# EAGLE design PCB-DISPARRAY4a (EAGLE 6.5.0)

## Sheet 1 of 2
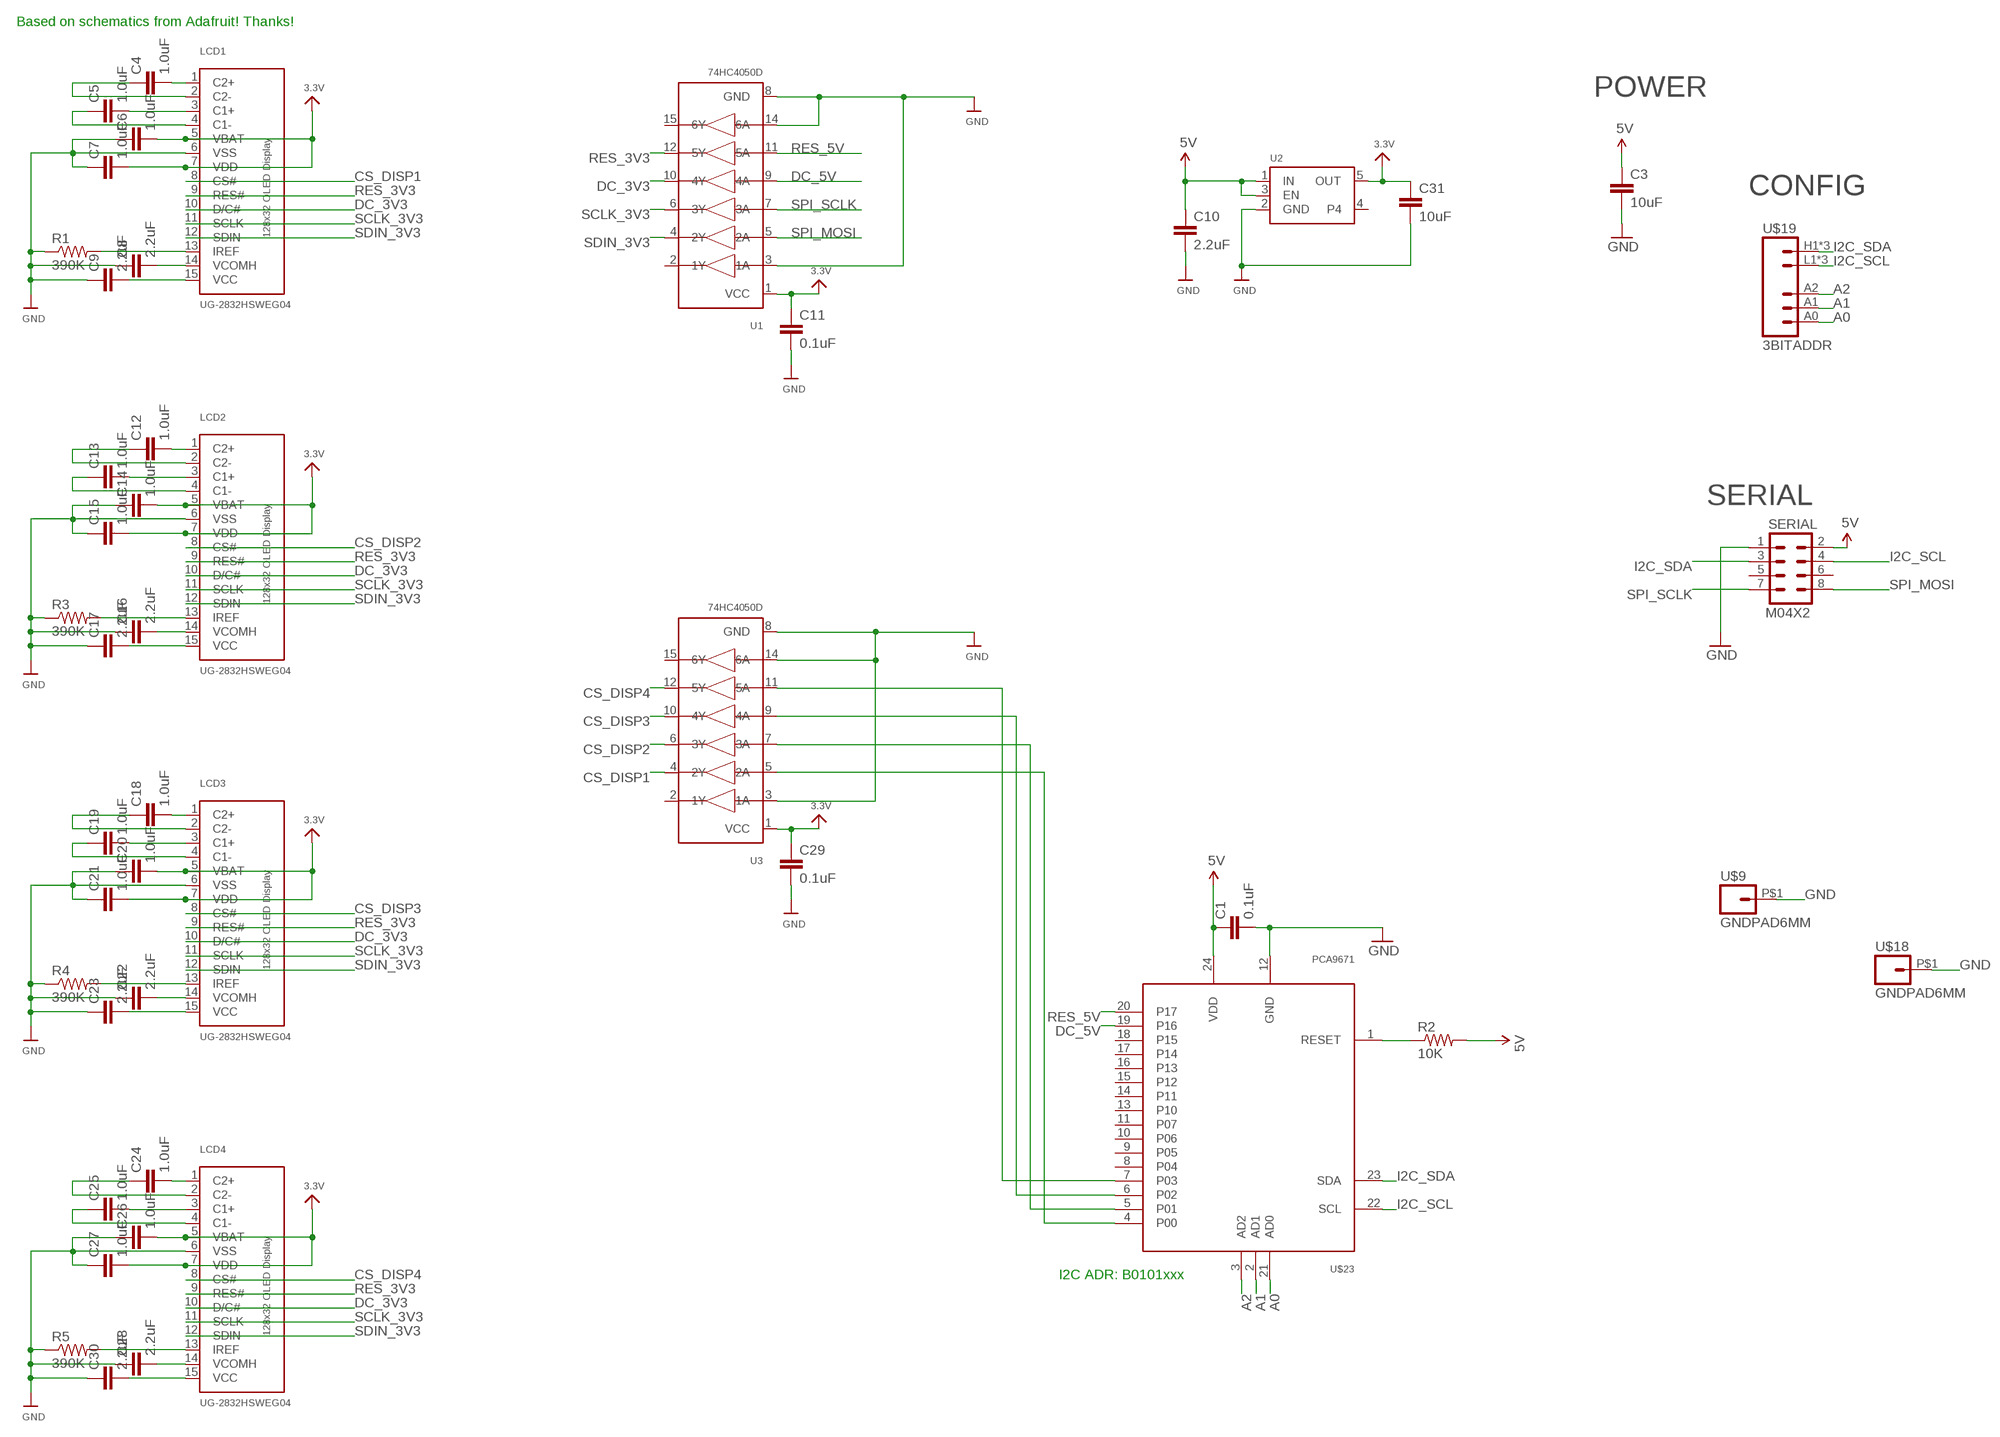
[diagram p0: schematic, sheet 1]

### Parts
C1  0.1uF  CAP0603-CAP  [0603-CAP]
C3  10uF  CAP0805  [0805]
C4  1.0uF  CAP0603-CAP  [0603-CAP]
C5  1.0uF  CAP0603-CAP  [0603-CAP]
C6  1.0uF  CAP0603-CAP  [0603-CAP]
C7  1.0uF  CAP0603-CAP  [0603-CAP]
C8  2.2uF  CAP0603-CAP  [0603-CAP]
C9  2.2uF  CAP0603-CAP  [0603-CAP]
C10  2.2uF  CAP0805  [0805]
C11  0.1uF  CAP0603-CAP  [0603-CAP]
C12  1.0uF  CAP0603-CAP  [0603-CAP]
C13  1.0uF  CAP0603-CAP  [0603-CAP]
C14  1.0uF  CAP0603-CAP  [0603-CAP]
C15  1.0uF  CAP0603-CAP  [0603-CAP]
C16  2.2uF  CAP0603-CAP  [0603-CAP]
C17  2.2uF  CAP0603-CAP  [0603-CAP]
C18  1.0uF  CAP0603-CAP  [0603-CAP]
C19  1.0uF  CAP0603-CAP  [0603-CAP]
C20  1.0uF  CAP0603-CAP  [0603-CAP]
C21  1.0uF  CAP0603-CAP  [0603-CAP]
C22  2.2uF  CAP0603-CAP  [0603-CAP]
C23  2.2uF  CAP0603-CAP  [0603-CAP]
C24  1.0uF  CAP0603-CAP  [0603-CAP]
C25  1.0uF  CAP0603-CAP  [0603-CAP]
C26  1.0uF  CAP0603-CAP  [0603-CAP]
C27  1.0uF  CAP0603-CAP  [0603-CAP]
C28  2.2uF  CAP0603-CAP  [0603-CAP]
C29  0.1uF  CAP0603-CAP  [0603-CAP]
C30  2.2uF  CAP0603-CAP  [0603-CAP]
C31  10uF  CAP0805  [0805]
LCD1  UG-2832HSWEG04  OLED_UG-2832HSWEG04WRAPAROUND  [UG-2832HSWEG04_WRAPAROUND]
LCD2  UG-2832HSWEG04  OLED_UG-2832HSWEG04WRAPAROUND  [UG-2832HSWEG04_WRAPAROUND]
LCD3  UG-2832HSWEG04  OLED_UG-2832HSWEG04WRAPAROUND  [UG-2832HSWEG04_WRAPAROUND]
LCD4  UG-2832HSWEG04  OLED_UG-2832HSWEG04WRAPAROUND  [UG-2832HSWEG04_WRAPAROUND]
R1  390K  RESISTOR0603-RES  [0603-RES]
R2  10K  RESISTOR0603-RES  [0603-RES]
R3  390K  RESISTOR0603-RES  [0603-RES]
R4  390K  RESISTOR0603-RES  [0603-RES]
R5  390K  RESISTOR0603-RES  [0603-RES]
SERIAL  M04X2  [2X4]
U1  74HC4050D  74HC4050DTSSOP16  [TSSOP16]
U2  VREG_SOT23-5  [SOT23-5]
U3  74HC4050D  74HC4050DTSSOP16  [TSSOP16]
U$9  GNDPAD6MM  [3.2MMPAD6MM]
U$18  GNDPAD6MM  [3.2MMPAD6MM]
U$19  3BITADDR  [3BITADDR]
U$23  PCA9671  [TSSOP24]

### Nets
3.3V [Power]: C6.2 C7.2 C11.1 C14.2 C15.2 C20.2 C21.2 C26.2 C27.2 C29.1 C31.1 LCD1.5(VBAT) LCD1.7(VDD) LCD2.5(VBAT) LCD2.7(VDD) LCD3.5(VBAT) LCD3.7(VDD) LCD4.5(VBAT) LCD4.7(VDD) U1.1(VCC) U2.5(OUT) U3.1(VCC)
5V [Power]: C1.1 C3.1 C10.1 R2.2 SERIAL.2 U2.1(IN) U2.3(EN) U$23.24(VDD)
A0: U$19.A0 U$23.21(AD0)
A1: U$19.A1 U$23.2(AD1)
A2: U$19.A2 U$23.3(AD2)
CS_DISP1: LCD1.8(CS#) U3.4(2Y)
CS_DISP2: LCD2.8(CS#) U3.6(3Y)
CS_DISP3: LCD3.8(CS#) U3.10(4Y)
CS_DISP4: LCD4.8(CS#) U3.12(5Y)
DC_3V3: LCD1.10(D/C#) LCD2.10(D/C#) LCD3.10(D/C#) LCD4.10(D/C#) U1.10(4Y)
DC_5V: U1.9(4A) U$23.19(P16)
GND [Power]: C1.2 C3.2 C6.1 C7.1 C8.1 C9.1 C10.2 C11.2 C14.1 C15.1 C16.1 C17.1 C20.1 C21.1 C22.1 C23.1 C26.1 C27.1 C28.1 C29.2 C30.1 C31.2 LCD1.6(VSS) LCD2.6(VSS) LCD3.6(VSS) LCD4.6(VSS) R1.1 R3.1 R4.1 R5.1 SERIAL.1 U1.3(1A) U1.8(GND) U1.14(6A) U2.2(GND) U3.3(1A) U3.8(GND) U3.14(6A) U$9.P$1 U$18.P$1 U$23.12(GND)
I2C_SCL: SERIAL.4 U$19.L1(GND) U$19.L2(GND) U$19.L3(GND) U$23.22(SCL)
I2C_SDA: SERIAL.3 U$19.H1(VCC) U$19.H2(VCC) U$19.H3(VCC) U$23.23(SDA)
N$1: R2.1 U$23.1(RESET)
N$2: C4.1 LCD1.2(C2-)
N$3: C4.2 LCD1.1(C2+)
N$4: C5.1 LCD1.4(C1-)
N$5: C12.1 LCD2.2(C2-)
N$6: C12.2 LCD2.1(C2+)
N$7: C5.2 LCD1.3(C1+)
N$8: LCD1.13(IREF) R1.2
N$9: C8.2 LCD1.14(VCOMH)
N$10: C13.1 LCD2.4(C1-)
N$11: C13.2 LCD2.3(C1+)
N$12: LCD2.13(IREF) R3.2
N$13: C16.2 LCD2.14(VCOMH)
N$14: C17.2 LCD2.15(VCC)
N$15: C18.1 LCD3.2(C2-)
N$16: C18.2 LCD3.1(C2+)
N$17: C19.1 LCD3.4(C1-)
N$18: C19.2 LCD3.3(C1+)
N$19: LCD3.13(IREF) R4.2
N$20: C22.2 LCD3.14(VCOMH)
N$21: C23.2 LCD3.15(VCC)
N$22: C24.1 LCD4.2(C2-)
N$23: C24.2 LCD4.1(C2+)
N$24: C25.1 LCD4.4(C1-)
N$25: C25.2 LCD4.3(C1+)
N$26: LCD4.13(IREF) R5.2
N$27: C28.2 LCD4.14(VCOMH)
N$28: C9.2 LCD1.15(VCC)
N$29: U3.5(2A) U$23.4(P00)
N$30: U3.7(3A) U$23.5(P01)
N$31: U3.9(4A) U$23.6(P02)
N$32: U3.11(5A) U$23.7(P03)
N$33: C30.2 LCD4.15(VCC)
RES_3V3: LCD1.9(RES#) LCD2.9(RES#) LCD3.9(RES#) LCD4.9(RES#) U1.12(5Y)
RES_5V: U1.11(5A) U$23.20(P17)
SCLK_3V3: LCD1.11(SCLK) LCD2.11(SCLK) LCD3.11(SCLK) LCD4.11(SCLK) U1.6(3Y)
SDIN_3V3: LCD1.12(SDIN) LCD2.12(SDIN) LCD3.12(SDIN) LCD4.12(SDIN) U1.4(2Y)
SPI_MOSI: SERIAL.8 U1.5(2A)
SPI_SCLK: SERIAL.7 U1.7(3A)
Unconnected: SERIAL.5 SERIAL.6 U1.2(1Y) U1.15(6Y) U2.4 U3.2(1Y) U3.15(6Y) U$23.8(P04) U$23.9(P05) U$23.10(P06) U$23.11(P07) U$23.13(P10) U$23.14(P11) U$23.15(P12) U$23.16(P13) U$23.17(P14) U$23.18(P15)

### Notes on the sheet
- Based on schematics from Adafruit! Thanks!
- POWER
- CONFIG
- SERIAL
- I2C ADR: B0101xxx

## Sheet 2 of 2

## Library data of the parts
C1 C3-C31 = SparkFun:CAP: Capacitor
LCD1-LCD4 = microbuilder:OLED_UG-2832HSWEG04: 128x32 SPI 0.91" Monochrome OLED Display
R1-R5 = SparkFun:RESISTOR: Resistor
SERIAL = SparkFun:M04X2
U1 U3 = SKAARHOJ:74HC4050D: 6-channel level shifter 74HC4050D - 2V-6V Supply Digikey: 74HC4050D,653-ND Mouser: 771-74HC4050D-T
U2 = microbuilder:VREG_SOT23-5: SOT23-5 Fixed Voltage Regulators To better organise some of the SOT23-5 fixed voltage regulators in this library, this new part was created. Part Current Out V Out V In V Dropout Digikey Part No. ADP121 150mA 3.3V 3.4-5.5V 0.09V @ 150mA ADP121-AUJZ33R7CT-ND ADP121 150mA 3.0V 3.1-5.5V 0.09V @ 150mA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
U$9 U$18 = SKAARHOJ:GNDPAD
U$19 = SKAARHOJ:3BITADDR
U$23 = SKAARHOJ:PCA9671

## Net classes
0 default: width 0.203 mm, drill 0.406 mm, clearance 0.152 mm
1 Power: width 0.406 mm, drill 0.61 mm, clearance 0.203 mm

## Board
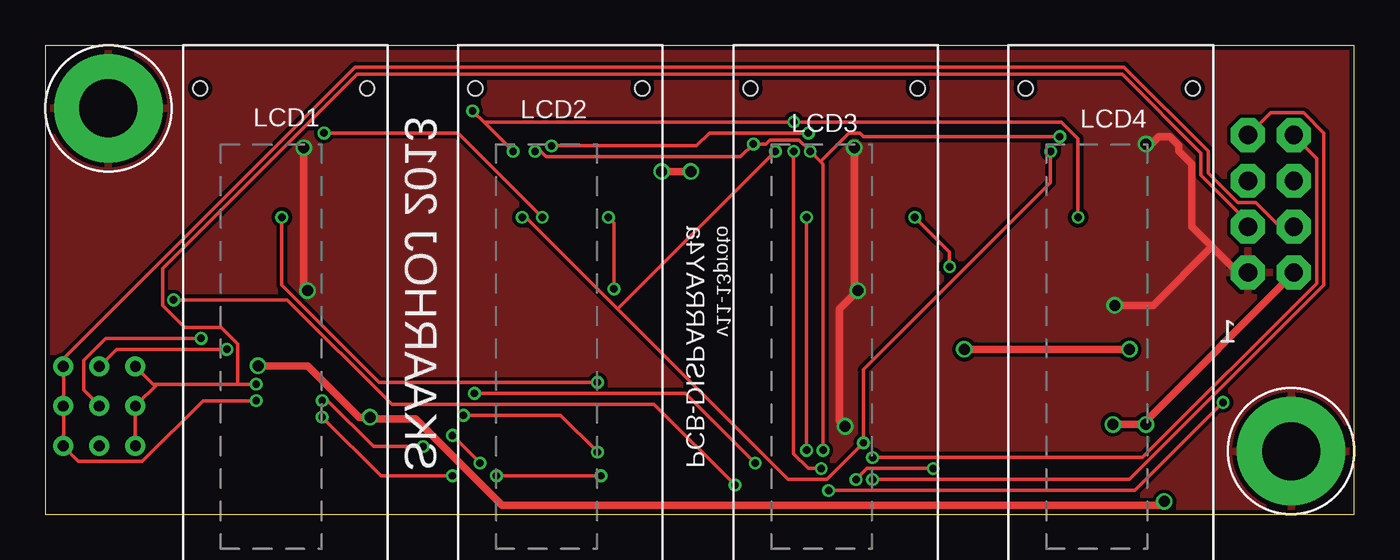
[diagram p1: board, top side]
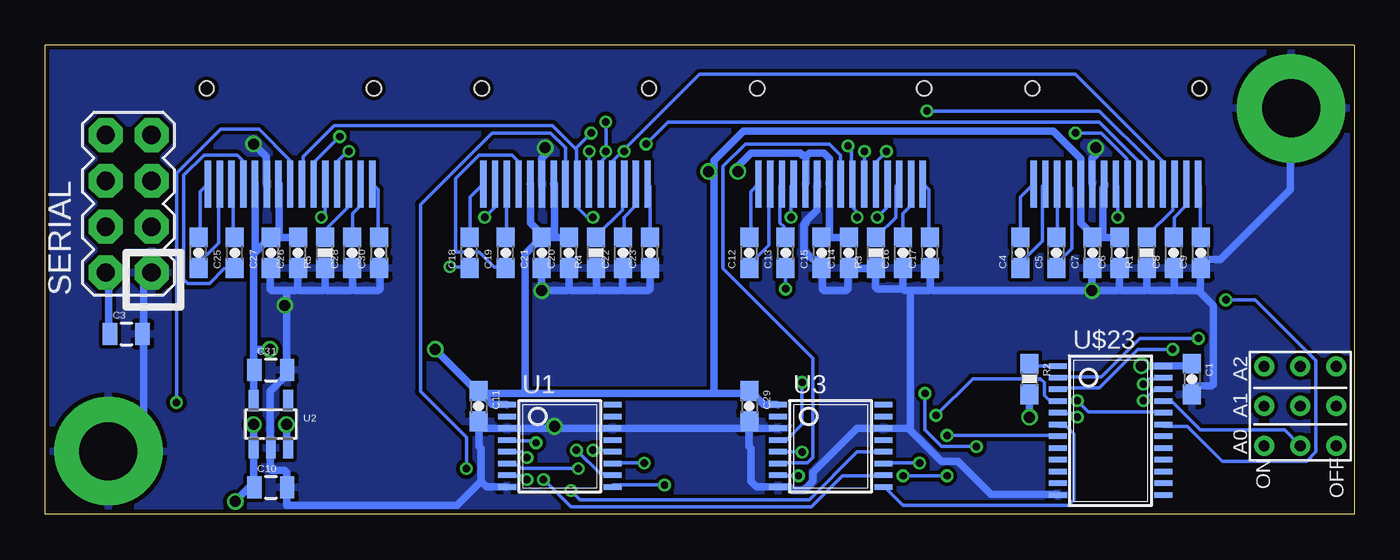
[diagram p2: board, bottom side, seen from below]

Size 72.5 x 26 mm. Coordinates in mm from the lower left corner, seen from the top.
Outline: 72.5,0 72.5,26 0,26 0,0 72.5,0
Copper layers (1*16): Top 0.035mm / dielectric 1.5mm / Bottom 0.035mm
Design rules "Fusion_eagle_rule_v1.1": minimum track width 6mil, minimum drill 12mil, track to track 6mil, track to pad 6mil, pad to pad 6mil, via to via 6mil, smd to smd 0mil, copper to edge 10mil, drill to drill 10mil, minimum pad ring 10mil, minimum via ring 6mil, stop-mask expansion 2mil, vias tented up to drill 100mil, thermal gap 10mil

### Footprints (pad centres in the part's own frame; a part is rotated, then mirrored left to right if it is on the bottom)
0603-CAP = smd 1.1 x 1: 1 -0.85,0; 2 0.85,0
0805 = smd 0.8 x 1.2: 1 -0.9,0; 2 0.9,0
UG-2832HSWEG04_WRAPAROUND = smd 2.6 x 0.35 bottom: 1 -7.7,-4.55; 2 -7.7,-3.9; 3 -7.7,-3.25; 4 -7.7,-2.6; 5 -7.7,-1.95; 6 -7.7,-1.3; 7 -7.7,-0.65; 8 -7.7,0; 9 -7.7,0.65; 10 -7.7,1.3; 11 -7.7,1.95; 12 -7.7,2.6; 13 -7.7,3.25; 14 -7.7,3.9; 15 -7.7,4.55 | hole 0.8: -2.4,4.625; -2.4,-4.625
0603-RES = smd 1.1 x 1: 1 -0.85,0; 2 0.85,0
2X4 = drill 1.016 pad 1.88 octagon: 1 -3.81,-1.27; 2 -3.81,1.27; 3 -1.27,-1.27; 4 -1.27,1.27; 5 1.27,-1.27; 6 1.27,1.27; 7 3.81,-1.27; 8 3.81,1.27
TSSOP16 = smd 0.305 x 0.991: 1 -3.575,-2.918; 2 -2.925,-2.918; 3 -2.275,-2.918; 4 -1.625,-2.918; 5 -0.975,-2.918; 6 -0.325,-2.918; 7 0.325,-2.918; 8 0.975,-2.918; 9 0.975,2.918; 10 0.325,2.918; 11 -0.325,2.918; 12 -0.975,2.918; 13 -1.625,2.918; 14 -2.275,2.918; 15 -2.925,2.918; 16 -3.575,2.918
SOT23-5 = smd 0.55 x 1.2: 1 -0.95,-1.3; 2 0,-1.3; 3 0.95,-1.3; 4 0.95,1.3; 5 -0.95,1.3
3.2MMPAD6MM = drill 3.2 pad 6: P$1 0,0
3BITADDR = drill 0.6: A0 -2.2,0; A1 0,0; A2 2.2,0; H1 -2.2,2; H2 0,2; H3 2.2,2; L1 -2.2,-2; L2 0,-2; L3 2.2,-2
TSSOP24 = smd 0.305 x 0.991: 1 -4.225,-2.918; 2 -3.575,-2.918; 3 -2.925,-2.918; 4 -2.275,-2.918; 5 -1.625,-2.918; 6 -0.975,-2.918; 7 -0.325,-2.918; 8 0.325,-2.918; 9 0.975,-2.918; 10 1.625,-2.918; 11 2.275,-2.918; 12 2.925,-2.918; 13 2.925,2.918; 14 2.275,2.918; 15 1.625,2.918; 16 0.975,2.918; 17 0.325,2.918; 18 -0.325,2.918; 19 -0.975,2.918; 20 -1.625,2.918; 21 -2.275,2.918; 22 -2.925,2.918; 23 -3.575,2.918; 24 -4.225,2.918

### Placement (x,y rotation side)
C1  9,7.5 270 bottom
C3  68,10 0 bottom
C4  18.5,14.5 90 bottom
C5  16.5,14.5 90 bottom
C6  13,14.5 90 bottom
C7  14.5,14.5 90 bottom
C8  10,14.5 90 bottom
C9  8.5,14.5 90 bottom
C10  60,1.5 0 bottom
C11  48.5,6 270 bottom
C12  33.5,14.5 90 bottom
C13  31.5,14.5 90 bottom
C14  28,14.5 90 bottom
C15  29.5,14.5 90 bottom
C16  25,14.5 90 bottom
C17  23.5,14.5 90 bottom
C18  49,14.5 90 bottom
C19  47,14.5 90 bottom
C20  43.5,14.5 90 bottom
C21  45,14.5 90 bottom
C22  40.5,14.5 90 bottom
C23  39,14.5 90 bottom
C24  64,14.5 90 bottom
C25  62,14.5 90 bottom
C26  58.5,14.5 90 bottom
C27  60,14.5 90 bottom
C28  55.5,14.5 90 bottom
C29  33.5,6 270 bottom
C30  54,14.5 90 bottom
C31  60,8 0 bottom
LCD1  13.21,26 90 top
LCD2  28.45,26 90 top
LCD3  43.69,26 90 top
LCD4  58.93,26 90 top
R1  11.5,14.5 90 bottom
R2  18,7.5 270 bottom
R3  26.5,14.5 90 bottom
R4  42,14.5 90 bottom
R5  57,14.5 90 bottom
SERIAL  67.88,17.21 90 bottom
U1  44,2.5 270 bottom
U2  60,5 0 bottom
U3  29,2.5 270 bottom
U$9  69,3.5 0 top
U$18  3.5,22.5 0 top
U$19  3,6 90 bottom
U$23  13.5,4 270 bottom

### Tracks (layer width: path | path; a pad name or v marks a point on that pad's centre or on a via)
3.3V  (via drill 0.61)
  Top 0.406: v35.76,19 v34.14,19 | v50.9,9.14 v60.05,9.14
  Bottom 0.406: U2.5 60.96,6.4 60.96,7.92 C31.1 60.96,8.13 60.96,9.14 | C26.2 58.52,15.34 59.94,15.34 C27.2 | C27.2 59.54,15.44 59.54,18.29 LCD4.7 | 60.96,9.14 60.96,14.43 60.76,14.63 | 60.76,14.63 60.15,15.24 C27.2 | LCD4.5 60.86,18.29 60.86,14.73 60.76,14.63 | 44.3,15.34 44.91,15.34 C21.2 | 44.3,15.34 43.59,15.34 C20.2 | 44.3,15.34 44.3,18.29 LCD3.7 | LCD3.5 45.62,18.29 45.62,16.15 45.01,15.54 C21.2 | C14.2 28.04,15.34 29.46,15.34 C15.2 29.06,15.44 29.06,18.29 LCD2.7 29.06,18.49 29.06,19.71 29.36,20.02 30.18,20.02 30.38,19.81 | 30.38,19.81 30.38,18.39 LCD2.5 | 13.92,15.34 14.43,15.34 C7.2 14.53,15.54 15.14,16.15 15.14,18.29 LCD1.5 15.14,18.49 15.14,19.71 16.66,21.23 33.83,21.23 35.46,19.61 35.46,19 | 13.92,15.34 C6.2 | 13.92,15.34 13.92,18.09 13.82,18.19 13.82,18.29 LCD1.7 | U3.1 32,6.1 32.72,6.1 33.43,6.81 C29.1 33.63,6.71 35.46,6.71 | U1.1 46.94,6.1 47.75,6.1 48.46,6.81 C11.1 | 45.92,6.71 48.16,6.71 C11.1 | 45.92,6.71 35.46,6.71 | 35.46,6.71 35.46,19 | v34.14,19 34.14,19.3 33.43,20.02 30.68,20.02 30.58,19.91 30.48,19.91 30.38,19.81 | 35.46,19 v35.76,19 | 45.92,6.71 45.92,14.43 45.11,15.24 C21.2 | v60.05,9.14 60.96,9.14 | v50.9,9.14 48.67,6.91 C11.1
5V  (via drill 0.61)
  Top 0.406: v11.79,8.23 14.53,8.23 17.37,5.38 v17.98,5.38 18.09,5.28 20.52,5.28 25.3,0.51 61.77,0.51 v61.98,0.71 | v59.13,4.98 60.76,4.98 60.86,5.08 | 60.86,5.08 69.09,13.31 SERIAL.2 | v60.96,4.98 60.86,5.08
  Bottom 0.406: C1.1 9.04,8.33 9.14,8.23 10.57,8.23 U$23.24 10.77,8.23 v11.79,8.23 | v17.98,5.38 17.98,6.6 R2.2 | v59.13,4.98 59.13,3.76 U2.3 | C3.1 68.99,10.06 68.99,13.21 69.09,13.31 SERIAL.2 | v60.96,4.98 60.96,3.86 U2.1 60.96,3.66 60.96,1.52 C10.1 61.16,1.52 v61.98,0.71
A0
  Bottom 0.203: U$23.21 10.57,6.2 10.06,6.2 8.53,4.67 3.86,4.67 3.05,3.86 U$19.A0
A1  (via drill 0.41)
  Top 0.203: v8.64,9.75 3.35,9.75 2.13,8.53 2.13,6.91 2.95,6.1 U$19.A1
  Bottom 0.203: v8.64,9.75 11.89,9.75 14.02,7.62 16.36,7.62 U$23.2
A2  (via drill 0.41)
  Top 0.203: v10.06,9.14 3.96,9.14 3.05,8.23 U$19.A2
  Bottom 0.203: v10.06,9.14 11.99,9.14 14.12,7.01 16.36,7.01 U$23.3
CS_DISP1  (via drill 0.41)
  Top 0.203: v30.58,7.32 18.49,7.32 13.11,12.7 v13.11,16.46
  Bottom 0.203: v30.58,7.32 30.58,4.98 31.39,4.17 31.9,4.17 U3.4 | v13.11,16.46 13.11,18.19 13.21,18.29 LCD1.8
CS_DISP2
  Bottom 0.203: LCD2.8 28.45,19.91 29.06,20.52 33.73,20.52 34.95,19.3 34.95,13.61 29.97,8.64 29.97,3.15 30.28,2.85 31.9,2.85 U3.6
CS_DISP3  (via drill 0.41)
  Top 0.203: v44.91,1.93 45.52,2.54 v49.17,2.54
  Bottom 0.203: v44.91,1.93 43.38,0.41 30.07,0.41 28.35,2.13 26.11,2.13 U3.10 | v49.17,2.54 49.17,4.27 51.71,6.81 51.71,17.17 47.75,21.13 44.5,21.13 43.69,20.32 LCD3.8
CS_DISP4  (via drill 0.41)
  Top 0.203: v43.38,1.32 60.35,1.32 v65.23,6.2
  Bottom 0.203: v43.38,1.32 42.88,0.81 30.18,0.81 27.53,3.45 26.11,3.45 U3.12 | v65.23,6.2 65.23,18.9 62.79,21.34 60.66,21.34 58.93,19.61 LCD4.8
DC_3V3  (via drill 0.41)
  Top 0.203: v43.08,3.56 43.08,19.41 42.93,19.56 | 42.93,19.56 v42.37,20.12 41.76,20.73 40.13,20.73 39.93,20.52 v39.22,20.52 38.51,19.81 27.74,19.81 27.43,20.12 v27.13,20.12 | v56.19,20.93 45.31,20.93 45.11,21.13 44.5,21.13 42.93,19.56
  Bottom 0.203: v43.08,3.56 41.76,2.23 41.15,2.23 U1.10 | v42.37,20.12 42.37,18.39 LCD3.10 | v39.22,20.52 38,21.74 14.12,21.74 11.99,19.61 11.99,18.39 LCD1.10 | v27.13,20.12 27.13,18.39 LCD2.10 | v56.19,20.93 57.61,19.51 57.61,18.39 LCD4.10
DC_5V  (via drill 0.41)
  Top 0.203: v7.11,11.89 13.41,11.89 19.2,6.1 33.73,6.1 v38.2,1.63
  Bottom 0.203: v7.11,11.89 5.49,11.89 2.13,8.53 2.13,3.45 2.64,2.95 7.32,2.95 9.25,4.88 10.57,4.88 U$23.19 | v38.2,1.63 41.05,1.63 U1.9
GND  (via drill 0.61)
  Top 0.406: v60.96,20.52 61.27,20.52 61.67,20.93 62.28,20.93 62.79,20.42 62.79,20.12 63.5,19.41 63.5,15.95 64.62,14.83 | 64.62,14.83 66.04,13.41 66.55,13.41 SERIAL.1 | v44.81,20.32 44.81,12.6 v45.01,12.39 43.99,11.38 43.99,5.18 v44.3,4.88 | v14.33,20.32 14.33,12.6 v14.53,12.39 | 64.62,14.83 61.37,11.58 v59.23,11.58
  Bottom 0.406: SERIAL.1 66.65,13.31 67.06,12.9 67.06,10.06 C3.2 67.06,9.86 67.06,5.49 68.99,3.56 U$9.P$1 | v60.96,20.52 60.25,19.81 60.25,18.39 LCD4.6 | 40.54,12.5 40.44,12.39 39.12,12.39 39.01,12.5 39.01,13.61 C23.1 | 40.54,12.5 40.54,13.61 C22.1 | 41.96,12.5 41.96,13.61 R4.1 | 41.96,12.5 41.86,12.39 40.64,12.39 40.54,12.5 | 43.48,12.5 43.48,13.61 C20.1 | 43.48,12.5 43.38,12.39 42.06,12.39 41.96,12.5 | 45.01,12.5 45.01,13.61 C21.1 | 45.01,12.5 44.91,12.39 43.59,12.39 43.48,12.5 | v44.81,20.32 44.81,19.91 45.01,19.71 45.01,18.39 LCD3.6 | v45.01,12.39 45.01,12.5 | 48.36,1.83 48.06,1.52 46.94,1.52 U1.8 | 48.36,1.83 48.36,3.66 48.46,3.76 48.46,5.08 C11.2 48.36,4.78 47.04,4.78 U1.3 46.84,4.78 44.3,4.78 | 44.3,4.78 41.15,4.78 U1.14 40.95,4.78 33.63,4.78 C29.2 | 55.47,12.5 55.37,12.39 54.05,12.39 53.95,12.5 53.95,13.61 C30.1 | 55.47,12.5 55.47,13.61 C28.1 | 57,12.5 57,13.61 R5.1 | 57,12.5 56.9,12.39 55.58,12.39 55.47,12.5 | 58.52,12.5 58.52,13.61 C26.1 | 58.52,12.5 58.42,12.39 57.1,12.39 57,12.5 | 59.13,12.39 58.62,12.39 58.52,12.5 | 59.13,12.39 59.94,12.39 60.05,12.5 60.05,13.61 C27.1 | 59.13,12.39 59.13,11.58 | 59.13,11.58 59.13,8.03 C31.2 59.03,7.82 60.05,6.81 60.05,3.86 U2.2 60.05,3.66 60.05,2.54 59.94,2.44 59.23,2.44 59.13,2.34 59.13,1.52 C10.2 59.13,1.32 59.13,0.51 49.68,0.51 48.36,1.83 | v44.3,4.88 44.3,4.78 | 8.64,12.39 8.53,12.5 8.53,13.61 C9.1 8.53,13.82 8.53,14.12 7.42,14.12 3.56,17.98 3.56,22.45 U$18.P$1 | 8.64,12.39 9.86,12.39 9.96,12.5 | 9.96,12.5 9.96,13.61 C8.1 | 8.64,12.39 7.82,11.58 7.82,7.21 7.92,7.11 9.04,7.11 9.04,6.71 C1.2 | 11.48,12.5 11.48,13.61 R1.1 | 11.48,12.5 11.38,12.39 10.06,12.39 9.96,12.5
  Bottom 0.406: 13.01,12.5 13.01,13.61 C6.1 | 13.01,12.5 12.9,12.39 11.58,12.39 11.48,12.5 | 14.53,12.5 14.53,13.61 C7.1 | 14.53,12.5 14.43,12.39 13.11,12.39 13.01,12.5 | v14.33,20.32 14.33,19.91 14.53,19.71 14.53,18.39 LCD1.6 | 14.53,12.5 v14.53,12.39 23.37,12.39 23.47,12.5 | 23.47,12.5 23.47,13.61 C17.1 | 23.47,12.5 23.57,12.39 24.59,12.39 | 24.59,12.39 24.89,12.39 24.99,12.5 | 24.99,12.5 24.99,13.61 C16.1 | 24.99,12.5 26.42,12.5 26.52,12.6 26.52,13.61 R3.1 26.72,13.61 27.84,13.61 C14.1 28.04,13.61 28.04,12.5 28.14,12.39 29.36,12.39 29.46,12.5 29.46,13.61 C15.1 29.46,13.82 29.46,14.12 29.97,14.12 30.48,14.63 30.48,16.05 30.38,16.15 30.38,16.26 29.77,16.87 29.77,18.29 LCD2.6 | C29.2 33.53,5.08 33.53,3.76 33.43,3.66 33.43,1.83 33.12,1.52 32,1.52 U3.8 31.8,1.52 31.29,1.52 31.09,1.32 30.48,1.32 29.97,1.83 29.97,2.34 27.53,4.78 26.21,4.78 U3.14 26.01,4.78 24.69,4.78 | U3.3 32,4.78 33.43,4.78 C29.2 | 24.69,4.78 22.86,2.95 21.95,2.95 20.12,1.12 16.46,1.12 U$23.12 | 24.59,12.39 24.59,4.88 24.69,4.78 | v59.23,11.58 59.13,11.58
  pour Top: 0,0 73,0 73,26 0,26
  pour Bottom: 0,0 73,0 73,26 0,26
I2C_SCL  (via drill 0.41)
  Top 0.203: v11.68,6.3 8.74,6.3 5.38,2.95 1.83,2.95 1.02,3.76 U$19.L1 1.02,3.86 1.02,5.99 U$19.L2 1.02,6.1 1.02,8.13 U$19.L3 1.02,8.23 1.02,8.64 17.17,24.79 59.74,24.79 64.41,20.12 64.41,18.9 66.04,17.27 67.06,17.27 68.38,15.95 69.09,15.95 SERIAL.4
  Bottom 0.203: v11.68,6.3 11.07,6.91 10.67,6.91 U$23.22
I2C_SDA  (via drill 0.41)
  Top 0.203: U$19.H1 4.98,3.86 4.98,5.99 U$19.H2 5.08,6.1 6.2,7.21 | 6.2,7.21 5.99,7.21 5.08,8.13 U$19.H3 | 6.2,7.21 10.67,7.21 | 10.67,7.21 v11.68,7.21 | 10.67,7.21 10.67,9.45 9.75,10.36 7.72,10.36 6.5,11.58 6.5,13.61 17.27,24.38 59.64,24.38 64.01,20.02 64.01,18.8 66.55,16.26 66.55,15.95 SERIAL.3
  Bottom 0.203: v11.68,7.21 11.38,7.52 10.67,7.52 U$23.23
N$1
  Bottom 0.203: U$23.1 16.46,8.23 17.88,8.23 17.98,8.33 R2.1
N$2
  Bottom 0.203: C4.1 18.49,13.72 18.49,13.92 17.27,15.14 17.27,18.19 17.17,18.29 LCD1.2
N$3
  Bottom 0.203: C4.2 18.49,15.44 18.49,17.58 17.78,18.29 LCD1.1
N$4
  Bottom 0.203: C5.1 16.46,13.72 16.46,13.92 15.65,14.73 15.65,18.09 15.85,18.29 LCD1.4
N$5
  Bottom 0.203: C12.1 33.43,13.72 33.43,13.92 32.41,14.94 32.41,18.29 LCD2.2
N$6
  Bottom 0.203: C12.2 33.43,15.44 33.43,17.88 33.02,18.29 LCD2.1
N$7
  Bottom 0.203: C5.2 16.46,15.44 16.46,18.29 LCD1.3
N$8
  Bottom 0.203: R1.2 11.48,15.44 10.06,16.87 10.06,18.29 LCD1.13
N$9
  Bottom 0.203: C8.2 9.96,15.44 9.96,16.46 9.35,17.07 9.35,18.29 LCD1.14
N$10  (via drill 0.41)
  Top 0.203: v31.5,12.5 31.5,16.15 v31.19,16.46
  Bottom 0.203: v31.5,12.5 31.5,13.61 C13.1 | v31.19,16.46 31.19,18.19 31.09,18.29 LCD2.4
N$11
  Bottom 0.203: C13.2 31.6,15.44 31.6,15.95 31.8,16.15 31.8,18.19 31.7,18.29 LCD2.3
N$12
  Bottom 0.203: R3.2 26.42,15.44 25.4,16.46 25.4,18.19 25.3,18.29 LCD2.13
N$13
  Bottom 0.203: C16.2 24.99,15.44 24.99,16.66 24.59,17.07 24.59,18.29 LCD2.14
N$14
  Bottom 0.203: C17.2 23.57,15.44 23.57,17.98 23.88,18.29 LCD2.15
N$15  (via drill 0.41)
  Top 0.203: v50.09,13.72 50.09,14.53 v48.16,16.46
  Bottom 0.203: v50.09,13.72 49.07,13.72 C18.1 | v48.16,16.46 47.65,16.97 47.65,18.29 LCD3.2
N$16
  Bottom 0.203: C18.2 48.97,15.44 48.97,17.58 48.26,18.29 LCD3.1
N$17
  Bottom 0.203: C19.1 47.04,13.72 47.65,13.72 48.46,14.53 49.68,14.53 49.78,14.63 49.78,18.59 48.46,19.91 46.63,19.91 46.33,19.61 46.33,18.39 LCD3.4
N$18
  Bottom 0.203: C19.2 46.94,15.44 46.94,18.29 LCD3.3
N$19
  Bottom 0.203: R4.2 41.96,15.44 40.54,16.87 40.54,18.29 LCD3.13
N$20
  Bottom 0.203: C22.2 40.44,15.44 40.44,16.46 39.83,17.07 39.83,18.29 LCD3.14
N$21
  Bottom 0.203: C23.2 39.01,15.44 39.01,18.19 39.12,18.29 LCD3.15
N$22
  Bottom 0.203: C24.1 63.91,13.72 63.91,14.02 62.89,15.04 62.89,18.29 LCD4.2
N$23
  Bottom 0.203: C24.2 63.91,15.44 63.91,17.88 63.5,18.29 LCD4.1
N$24
  Bottom 0.203: C25.1 62.08,13.61 62.59,13.61 63.4,12.8 64.62,12.8 64.82,13.01 64.82,18.8 63.7,19.91 61.87,19.91 61.57,19.61 61.57,18.39 LCD4.4
N$25
  Bottom 0.203: C25.2 62.08,15.44 62.08,18.29 LCD4.3
N$26
  Bottom 0.203: R5.2 57,15.44 57,15.75 55.78,16.97 55.78,18.29 LCD4.13
N$27
  Bottom 0.203: C28.2 55.47,15.44 55.47,16.66 55.07,17.07 55.07,18.29 LCD4.14
N$28
  Bottom 0.203: C9.2 8.53,15.44 8.53,18.19 8.64,18.29 LCD1.15
N$29  (via drill 0.41)
  Top 0.203: v23.16,5.49 28.55,5.49 v30.58,3.45
  Bottom 0.203: v23.16,5.49 21.13,7.52 17.37,7.52 17.17,7.32 17.17,6.6 16.87,6.3 16.46,6.3 U$23.4 | v30.58,3.45 31.9,3.45 U3.5
N$30  (via drill 0.41)
  Top 0.203: v15.34,5.38 18.59,2.13 v22.55,2.13 | v30.79,2.13 v24.99,2.13
  Bottom 0.203: v15.34,5.38 15.54,5.59 16.36,5.59 U$23.5 | v24.99,2.13 v22.55,2.13 | v30.79,2.13 31.9,2.13 U3.7
N$31
  Bottom 0.203: U$23.6 16.36,4.88 15.95,4.88 15.54,4.47 15.54,0.81 15.85,0.51 24.99,0.51 26.01,1.52 U3.9
N$32  (via drill 0.41)
  Top 0.203: v24.08,2.85 v22.55,4.37
  Bottom 0.203: v22.55,4.37 16.46,4.37 U$23.7 | v24.08,2.85 26.01,2.85 U3.11
N$33
  Bottom 0.203: C30.2 54.05,15.44 54.05,17.98 54.36,18.29 LCD4.15
RES_3V3  (via drill 0.41)
  Top 0.203: v15.44,21.13 22.86,21.13 v27.53,16.46 | v42.16,16.46 v42.16,3.56 | v28.04,20.42 36.07,20.42 36.78,21.13 v42.27,21.13
  Bottom 0.203: v15.44,21.13 14.02,21.13 12.6,19.71 12.6,18.39 LCD1.9 | v27.53,16.46 27.53,16.76 27.74,16.97 27.74,18.29 LCD2.9 27.84,18.39 27.84,20.22 v28.04,20.42 | v42.16,3.56 41.15,3.56 U1.12 | v42.16,16.46 42.47,16.46 42.98,16.97 42.98,18.29 LCD3.9 43.08,18.39 43.08,20.22 43.13,20.27 | 43.13,20.27 44.4,21.54 56.49,21.54 58.22,19.81 58.22,18.39 LCD4.9 | 43.13,20.27 v42.27,21.13
RES_5V  (via drill 0.41)
  Top 0.203: v15.34,6.3 15.65,6.3 18.19,3.76 v20.93,3.76 | v23.77,6.71 35.46,6.71 v39.32,2.85
  Bottom 0.203: v15.34,6.3 14.73,5.69 10.67,5.69 U$23.20 | v20.93,3.76 22.86,3.76 23.77,4.67 v23.77,6.71 | v39.32,2.85 41.05,2.85 U1.11
SCLK_3V3  (via drill 0.41)
  Top 0.203: v42.98,2.54 42.27,2.54 41.45,3.35 v41.45,20.12 | v25.91,20.12 24.33,21.69 | 24.33,21.69 v23.67,22.35 | v57.2,16.46 57.2,20.83 56.29,21.74 v41.45,21.74 24.38,21.74 24.33,21.69
  Bottom 0.203: v42.98,2.54 46.13,2.54 46.33,2.74 46.84,2.74 U1.6 | LCD3.11 41.66,18.39 41.66,19.61 41.45,19.81 v41.45,20.12 v41.45,21.74 | v23.67,22.35 14.12,22.35 11.28,19.51 11.28,18.39 LCD1.11 | v25.91,20.12 26.42,19.61 26.42,18.39 LCD2.11 | v57.2,16.46 57,16.66 57,18.29 LCD4.11
SDIN_3V3  (via drill 0.41)
  Top 0.203: v55.68,20.12 55.68,18.39 45.31,8.03 v45.31,3.96 43.28,1.93 41.15,1.93 31.7,11.38 | v26.42,16.46 26.62,16.46 31.7,11.38 | 31.7,11.38 v40.44,20.12
  Bottom 0.203: 40.49,20.17 41.05,19.61 41.05,18.39 LCD3.12 | 40.49,20.17 36.27,24.38 15.44,24.38 10.67,19.61 10.67,18.39 LCD1.12 | v45.31,3.96 45.41,4.06 46.84,4.06 U1.4 | v55.68,20.12 55.88,19.91 55.98,19.91 56.29,19.61 56.29,18.39 LCD4.12 | v26.42,16.46 25.91,16.97 25.91,18.29 LCD2.12 | v40.44,20.12 40.49,20.17
SPI_MOSI  (via drill 0.41)
  Top 0.203: v45.82,3.15 60.76,3.15 70.41,12.8 70.41,19.71 69.19,20.93 SERIAL.8
  Bottom 0.203: v45.82,3.15 46.13,3.45 46.84,3.45 U1.5
SPI_SCLK  (via drill 0.41)
  Top 0.203: v45.82,1.93 60.05,1.93 70.81,12.7 70.81,21.13 69.7,22.25 67.87,22.25 66.65,21.03 SERIAL.7
  Bottom 0.203: v45.82,1.93 46.02,2.13 46.84,2.13 U1.7

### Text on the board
_tsilk: SKAARHOJ 2013 | PCB-DISPARRAY4a | v11-13proto | 1

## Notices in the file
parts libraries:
SparkFun: Licensing: CC v3.0 Share-Alike You are welcome to use this library for commercial purposes.
